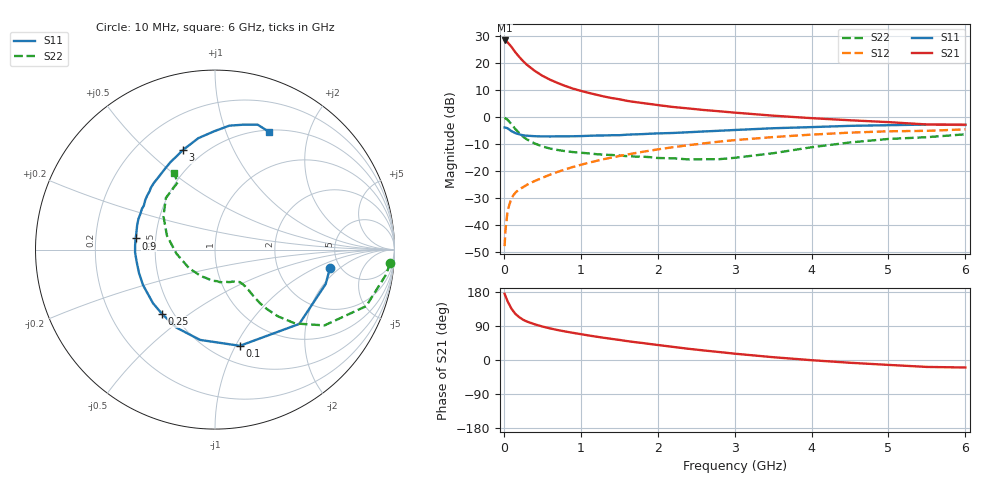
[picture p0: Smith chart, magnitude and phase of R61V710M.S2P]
! SIEMENS Small Signal Semiconductors
! BFR193
! Si NPN RF Bipolar Junction Transistor in SOT23
! VCE = 1.75 V  IC = 10 mA
! Common Emitter S-Parameters:  May  1996
# GHz  S  MA  R  50
!  f  S11  S21  S12  S22
! GHz  MAG  ANG  MAG  ANG  MAG  ANG  MAG  ANG
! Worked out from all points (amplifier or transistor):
!   36 points, 10 MHz to 6 GHz, reference 50 ohm
!   highest |S21| = 28.5 dB at 10 MHz (marker M1)
!   |S21| within 3 dB of that: start of sweep to 114.9 MHz
!   unconditionally stable (mu >= 1): 726.6 MHz to 1.954 GHz
!   at 250 MHz: K = 0.66, MSG = 23.4 dB, |S12| = -25.9 dB
!   at 1.4 GHz: K = 1.04, MAG = 9.8 dB, |S12| = -14.9 dB
!   at 6 GHz: K = 0.96, MSG = 0.9 dB, |S12| = -4.5 dB
!   S11 on the Smith chart (normalised r, x): 10 MHz: 4.17, -1.45; 100 MHz: 0.67, -1.04; 250 MHz: 0.43, -0.40; 900 MHz: 0.38, +0.06; 3 GHz: 0.39, +0.65; 6 GHz: 0.52, +1.42
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0.01  0.649 -8.9  26.56 174.7  0.0041 85.6  0.9803 -4.4
0.02  0.6457 -17.3  26.06 169.1  0.0078 85.5  0.9604 -8.7
0.05  0.6261 -41.4  24.43 154.4  0.019 71.5  0.8993 -20.5
0.1  0.5536 -75.5  20.12 135.1  0.0322 62.0  0.742 -34.7
0.15  0.51 -99.4  16.02 121.8  0.0403 56.3  0.6065 -42.7
0.2  0.4849 -116.4  13.17 113.0  0.0463 54.8  0.5103 -46.7
0.25  0.4642 -129.5  11.01 106.3  0.0508 54.3  0.4382 -48.9
0.3  0.4566 -139.2  9.405 101.4  0.0562 55.4  0.3897 -50.0
0.4  0.4472 -153.7  7.286 94.3  0.066 57.0  0.3283 -50.4
0.5  0.443 -163.1  5.904 88.4  0.0757 58.9  0.289 -50.3
0.6  0.4418 -171.4  4.986 83.4  0.0865 60.4  0.2641 -50.6
0.7  0.4457 -178.1  4.327 79.0  0.0975 61.4  0.2481 -51.2
0.9  0.4461 172.0  3.398 71.6  0.1204 62.2  0.227 -52.8
1.1  0.4549 162.4  2.845 64.8  0.1438 62.1  0.215 -56.9
1.3  0.461 154.5  2.436 58.6  0.1679 61.2  0.2028 -61.2
1.6  0.4772 144.4  2.022 50.0  0.204 59.1  0.1909 -70.5
2.2  0.513 127.5  1.554 34.6  0.2793 53.0  0.1742 -95.1
3  0.5822 108.1  1.222 16.7  0.378 41.8  0.1778 -144.1
3.5  0.6278 98.5  1.074 7.4  0.4307 34.0  0.2161 -174.1
4.5  0.6952 83.4  0.882 -7.3  0.5206 19.0  0.3423 147.0
5.5  0.7353 71.1  0.737 -18.3  0.5618 3.8  0.4286 118.9
6  0.7222 65.5  0.729 -19.8  0.5983 -0.7  0.4849 118.3
